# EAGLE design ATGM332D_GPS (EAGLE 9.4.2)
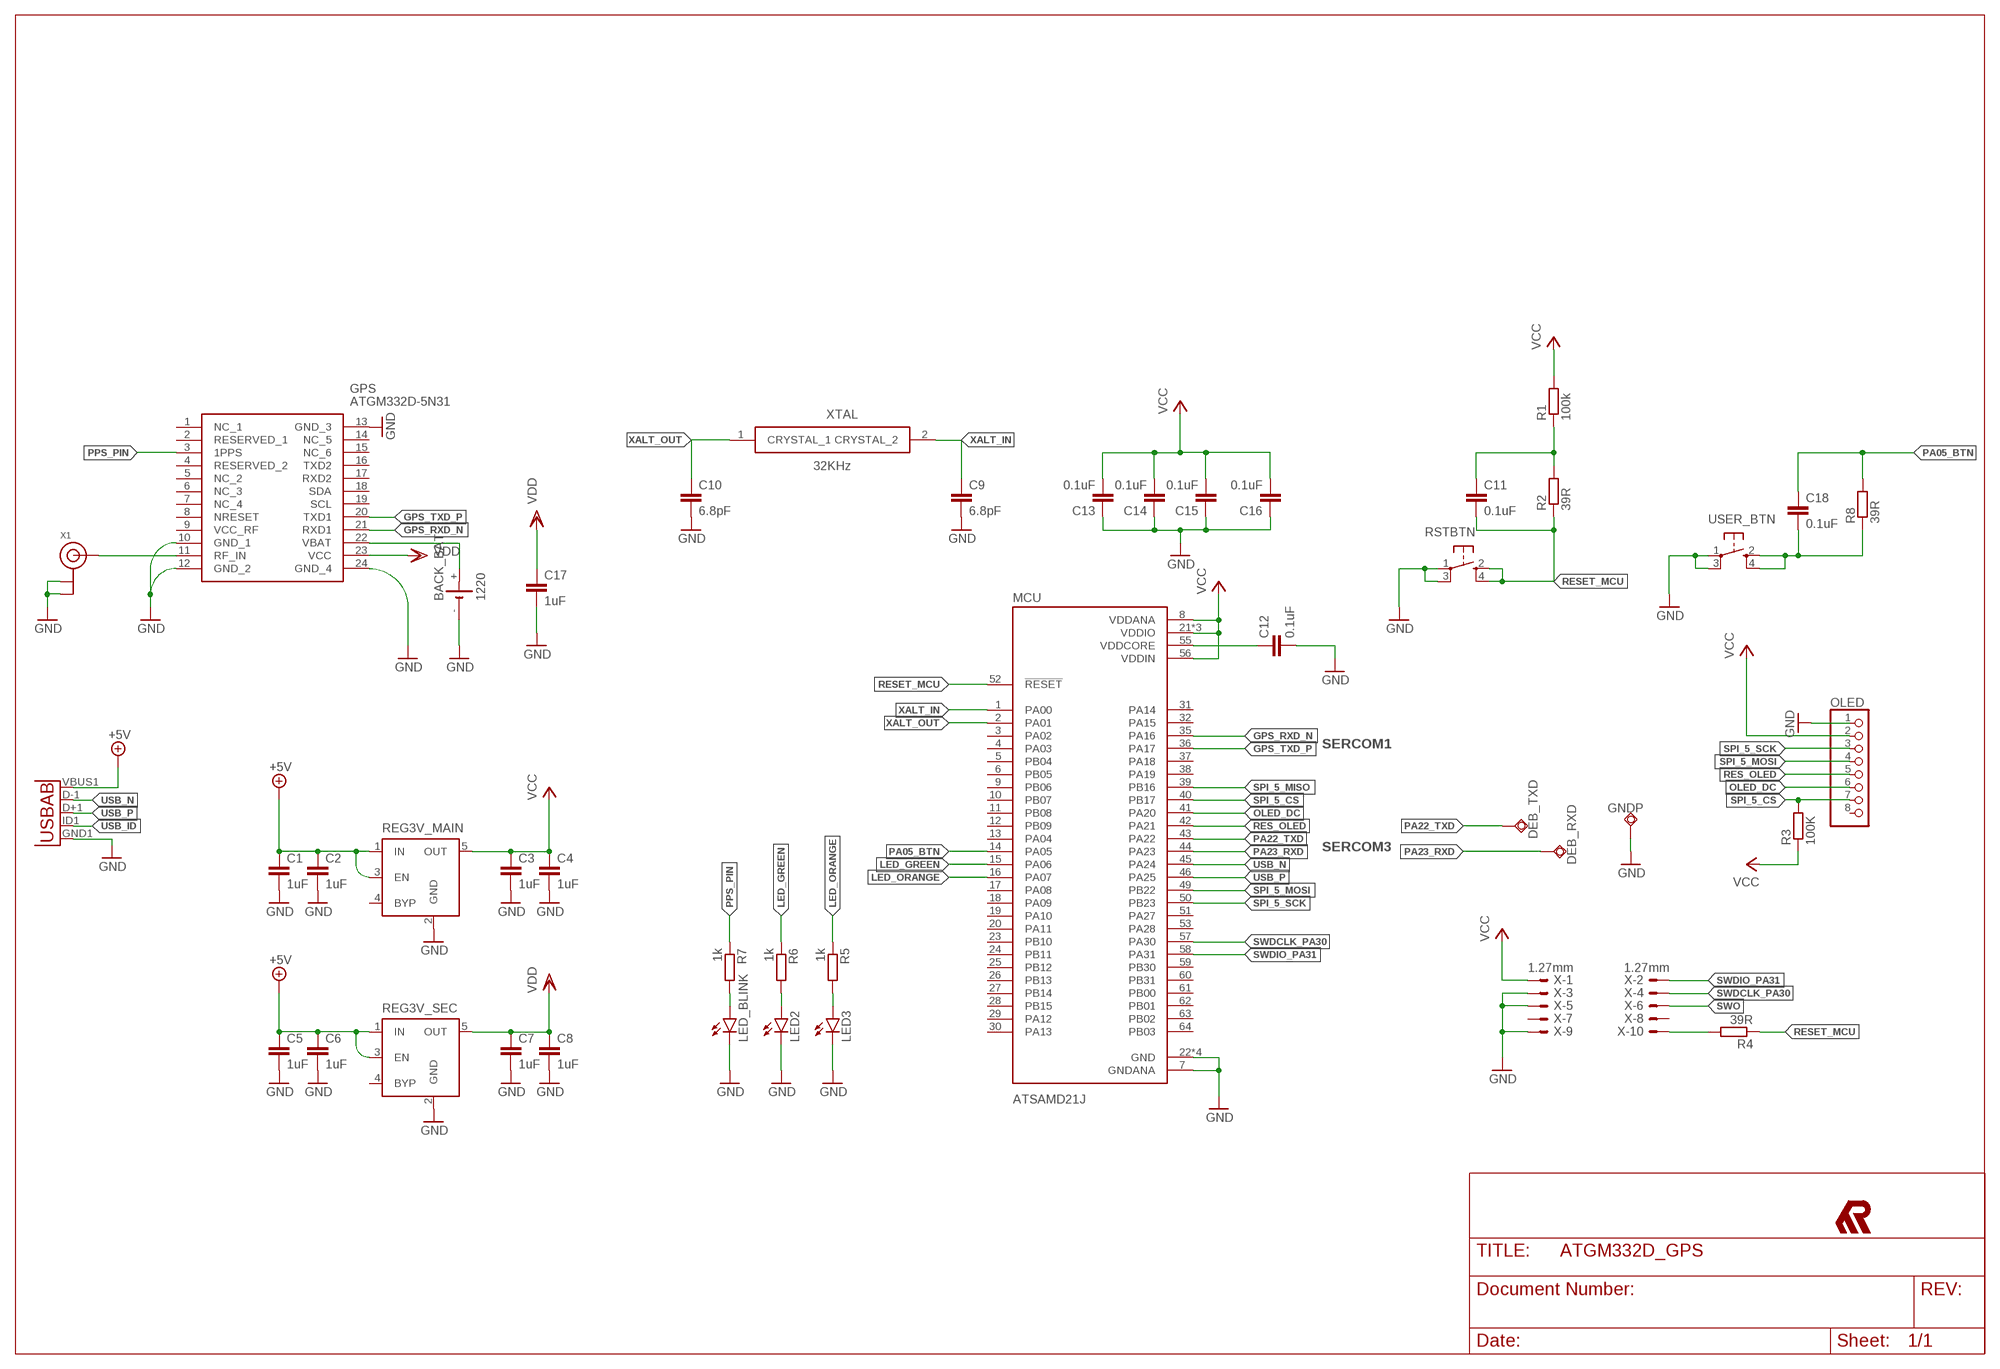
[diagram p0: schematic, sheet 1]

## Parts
BACK_BAT  1220  CH291-1220LF  [CH291-1220LF]
C1  1uF  C-EUC0805  [C0805]
C2  1uF  C-EUC0805  [C0805]
C3  1uF  C-EUC0805  [C0805]
C4  1uF  C-EUC0805  [C0805]
C5  1uF  C-EUC0805  [C0805]
C6  1uF  C-EUC0805  [C0805]
C7  1uF  C-EUC0805  [C0805]
C8  1uF  C-EUC0805  [C0805]
C9  6.8pF  C-EUC0603  [C0603]
C10  6.8pF  C-EUC0603  [C0603]
C11  0.1uF  C-EUC0603  [C0603]
C12  0.1uF  C-EUC0603  [C0603]
C13  0.1uF  C-EUC0603  [C0603]
C14  0.1uF  C-EUC0603  [C0603]
C15  0.1uF  C-EUC0603  [C0603]
C16  0.1uF  C-EUC0603  [C0603]
C17  1uF  C-EUC0805  [C0805]
C18  0.1uF  C-EUC0603  [C0603]
DEB_RXD  TPSQTP18R  [TP18R]
DEB_TXD  TPSQTP18R  [TP18R]
GNDP  TPSQTP18R  [TP18R]
GPS  ATGM332D-5N31  [ATGM332D5N31]
LED2  LEDCHIP-LED0603  [CHIP-LED0603]
LED3  LEDCHIP-LED0603  [CHIP-LED0603]
LED_BLINK  LEDCHIP-LED0603  [CHIP-LED0603]
MCU  ATSAMD21J  ATSAMD21J18A-AU  [QFP80P1600X1600X120-64N]
OLED  PINHD-1X8  [1X08]
R1  100k  R-EU_R0603  [R0603]
R2  39R  R-EU_R0603  [R0603]
R3  100K  R-EU_R0603  [R0603]
R4  39R  R-EU_R0603  [R0603]
R5  1k  R-EU_R0603  [R0603]
R6  1k  R-EU_R0603  [R0603]
R7  1k  R-EU_R0603  [R0603]
R8  39R  R-EU_R0603  [R0603]
REG3V_MAIN  MIC5219XX  [SOT23-5]
REG3V_SEC  MIC5219XX  [SOT23-5]
RSTBTN  SPST_TACT-KMR2  [KMR2]
U$2  MR_SMALL_SIZE12  [MR_SMALL_12MM]
USB  MICRO_USB_B  [USB-MICRO-SMD]
USER_BTN  SPST_TACT-KMR2  [KMR2]
X  1.27mm  1365-10  [1365-10]
X1  ANTENNA_U.FL  [U.FL]
XTAL  32KHz  SMD-3215_2P32.768KHZ12.5PF10PP  [SMD3215_2P32768KHZ125PF10PPM]

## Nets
+5V: C1.1 C2.1 C5.1 C6.1 REG3V_MAIN.1(IN) REG3V_MAIN.3(EN) REG3V_SEC.1(IN) REG3V_SEC.3(EN) USB.VBUS1(VBUS)
GND: BACK_BAT.- C1.2 C2.2 C3.2 C4.2 C5.2 C6.2 C7.2 C8.2 C9.2 C10.2 C12.2 C13.1 C14.1 C15.1 C16.1 C17.2 GNDP.TP GPS.10(GND_1) GPS.12(GND_2) GPS.13(GND_3) GPS.24(GND_4) LED2.C LED3.C LED_BLINK.C MCU.7(GNDANA) MCU.22(GND) MCU.33(GND) MCU.47(GND) MCU.54(GND) OLED.1 REG3V_MAIN.2(GND) REG3V_SEC.2(GND) RSTBTN.1(P) RSTBTN.3(P1) USB.GND1(GND) USER_BTN.1(P) USER_BTN.3(P1) X1.1(GND) X1.2(GND) X.3 X.5 X.9
GPS_RXD_N: GPS.21(RXD1) MCU.35(PA16)
GPS_TXD_P: GPS.20(TXD1) MCU.36(PA17)
LED_GREEN: MCU.15(PA06) R6.1
LED_ORANGE: MCU.16(PA07) R5.1
N$1: R4.2 X.10
N$2: LED_BLINK.A R7.2
N$3: LED2.A R6.2
N$4: LED3.A R5.2
N$5: C18.2 R8.1 USER_BTN.2(S) USER_BTN.4(S1)
N$8: BACK_BAT.+ GPS.22(VBAT)
N$9: GPS.11(RF_IN) X1.3(SIGNAL)
N$10: C11.1 R1.1 R2.2
OLED_DC: MCU.41(PA20) OLED.6
PA05_BTN: C18.1 MCU.14(PA05) R8.2
PA22_TXD: DEB_TXD.TP MCU.43(PA22)
PA23_RXD: DEB_RXD.TP MCU.44(PA23)
PPS_PIN: GPS.3(1PPS) R7.1
RES_OLED: MCU.42(PA21) OLED.5
RESET_MCU: C11.2 MCU.52(!RESET) R2.1 R4.1 RSTBTN.2(S) RSTBTN.4(S1)
SPI_5_CS: MCU.40(PB17) OLED.7 R3.2
SPI_5_MISO: MCU.39(PB16)
SPI_5_MOSI: MCU.49(PB22) OLED.4
SPI_5_SCK: MCU.50(PB23) OLED.3
SWDCLK_PA30: MCU.57(PA30) X.4
SWDIO_PA31: MCU.58(PA31) X.2
SWO: X.6
USB_ID: USB.ID1(USBID)
USB_N: MCU.45(PA24) USB.D-1(D-)
USB_P: MCU.46(PA25) USB.D+1(D+)
VCC: C3.1 C4.1 C13.2 C14.2 C15.2 C16.2 MCU.8(VDDANA) MCU.21(VDDIO) MCU.34(VDDIO) MCU.48(VDDIO) MCU.56(VDDIN) OLED.2 R1.2 R3.1 REG3V_MAIN.5(OUT) X.1
VCORE: C12.1 MCU.55(VDDCORE)
VDD: C7.1 C8.1 C17.1 GPS.23(VCC) REG3V_SEC.5(OUT)
XALT_IN: C9.1 MCU.1(PA00) XTAL.2(CRYSTAL_2)
XALT_OUT: C10.1 MCU.2(PA01) XTAL.1(CRYSTAL_1)
Unconnected: GPS.1(NC_1) GPS.2(RESERVED_1) GPS.4(RESERVED_2) GPS.5(NC_2) GPS.6(NC_3) GPS.7(NC_4) GPS.8(NRESET) GPS.9(VCC_RF) GPS.14(NC_5) GPS.15(NC_6) GPS.16(TXD2) GPS.17(RXD2) GPS.18(SDA) GPS.19(SCL) MCU.3(PA02) MCU.4(PA03) MCU.5(PB04) MCU.6(PB05) MCU.9(PB06) MCU.10(PB07) MCU.11(PB08) MCU.12(PB09) MCU.13(PA04) MCU.17(PA08) MCU.18(PA09) MCU.19(PA10) MCU.20(PA11) MCU.23(PB10) MCU.24(PB11) MCU.25(PB12) MCU.26(PB13) MCU.27(PB14) MCU.28(PB15) MCU.29(PA12) MCU.30(PA13) MCU.31(PA14) MCU.32(PA15) MCU.37(PA18) MCU.38(PA19) MCU.51(PA27) MCU.53(PA28) MCU.59(PB30) MCU.60(PB31) MCU.61(PB00) MCU.62(PB01) MCU.63(PB02) MCU.64(PB03) OLED.8 REG3V_MAIN.4(BYP) REG3V_SEC.4(BYP) X.7 X.8

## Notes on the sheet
- SERCOM1
- SERCOM3

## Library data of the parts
BACK_BAT = battery:CH291-1220LF: Battery Holder, SMT, 12mm
C1-C18 = rcl:C-EU: CAPACITOR, European symbol; SPICEPREFIX: C
DEB_RXD DEB_TXD GNDP = testpad:TPSQ: Test pad
GPS = ATGM332D-5N31:ATGM332D-5N31: Communication Modules/GNSS Modules 12.2x16x2.4mm Source: Datasheet; DESCRIPTION: Communication Modules/GNSS Modules 12.2x16x2.4mm; HEIGHT: 2.6mm; MANUFACTURER_NAME: ZHONGKEWEI; MANUFACTURER_PART_NUMBER: ATGM332D-5N31
LED2 LED3 LED_BLINK = led:LED: LED
MCU = ATSAMD21J18A-AU:ATSAMD21J18A-AU: 256kB Flash, 32kB SRAM, SERCOM, USB - 64TQFP IND TEMP, GREEN, 1.6-3.6V, 48MHz/ TQFP (A); DESCRIPTION: SAMD21J Series 256 kB Flash 32 kB RAM 48 MHz 32-Bit Microcontroller - TQFP-64; DIGI-KEY_PART_NUMBER: ATSAMD21J18A-AU-ND; DIGI-KEY_PURCHASE_URL: https://www.digikey.com/product-detail/en/microchip-technology/ATSAMD21J18A-AU/ATSAMD21J18A-AU-ND/4935901?utm_source=snapeda&utm_medium=aggregator&utm_campaign=symbol; MF: Microchip; MP: ATSAMD21J18A-AU; PACKAGE: TQFP-64 Microchip
OLED = pinhead:PINHD-1X8: PIN HEADER
R1-R8 = rcl:R-EU_: RESISTOR, European symbol; SPICEPREFIX: R
REG3V_MAIN REG3V_SEC = v-reg-micrel:MIC5219XX: VOLTAGE REGULATOR; OC_FARNELL: unknown; OC_NEWARK: unknown
RSTBTN USER_BTN = adafruit:SPST_TACT: SMT 6mm switch, EVQQ2 series http://www.ladyada.net/library/eagle
U$2 = Rawashdeh_Eagle_Logo:MR_SMALL_SIZE: MR Mohannad Rawashdeh Logo 7,12 mm
USB = Rawashdeh_Eagle_Connector:MICRO_USB_B: USB - micro B USB 2.0 Receptacle Connector 5 Position Surface Mount, Right Angle; Through Hole Manf. # 10118194-0001LF
X = con-leotronics:1365-10: DUAL ROW STRAIGHT HEADER 1364 SERIES. 1.27mm x 1.27mm. Without Fixing Post. SMT Source: http://www.leotronics.co.uk/Conexcon/Data%20Sheets/sec.%20A/1364ing.pdf; OC_FARNELL: unknown; OC_NEWARK: unknown
X1 = adafruit:ANTENNA_U.FL: U.FL Antenna Connector
XTAL = SMD-3215_2P32.768KHZ12.5PF10PP:SMD-3215_2P32.768KHZ12.5PF10PP: SMD Crystal Resonators 32.768KHz +/-10ppm SMD-3215_2P RoHS; DESCRIPTION: SMD Crystal Resonators 32.768KHz +/-10ppm SMD-3215_2P RoHS; HEIGHT: 0.8mm; LCSC_PART_NUMBER: C164062; LCSC_PRICE-STOCK: https://lcsc.com/product-detail/SMD-Crystal-Resonators_Zhejiang-Abel-Elec-SMD-3215-2P32-768KHZ12-5PF10PPM_C164062.html; MANUFACTURER_NAME: Zhejiang Abel Elec; MANUFACTURER_PART_NUMBER: SMD-3215_2P32.768KHZ12.5PF10PPM

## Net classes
1 VCC: width 0.203 mm, clearance 0.152 mm
2 VDD: width 0.203 mm, clearance 0.152 mm

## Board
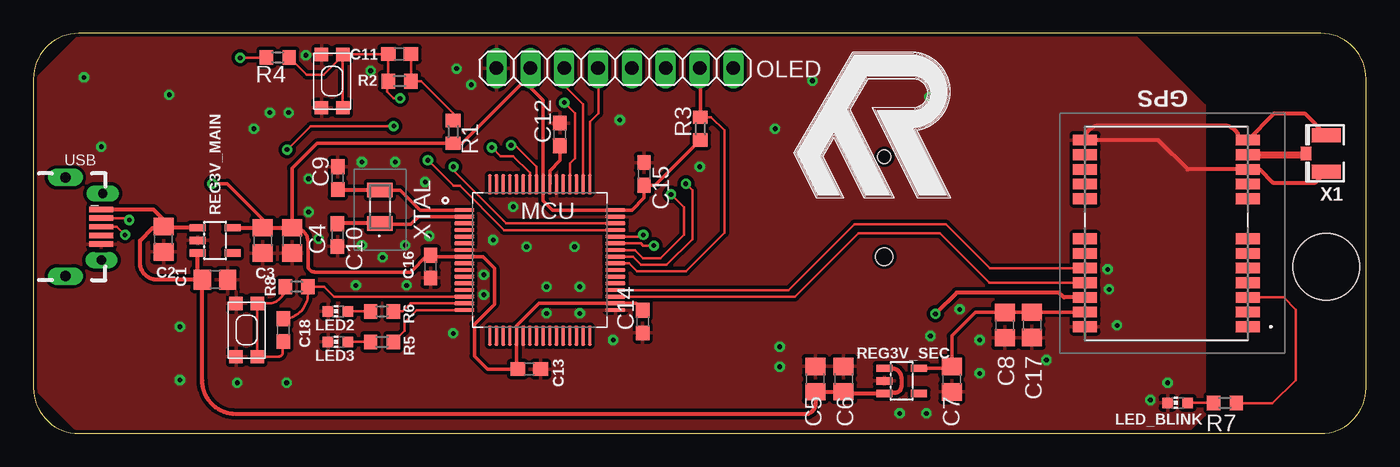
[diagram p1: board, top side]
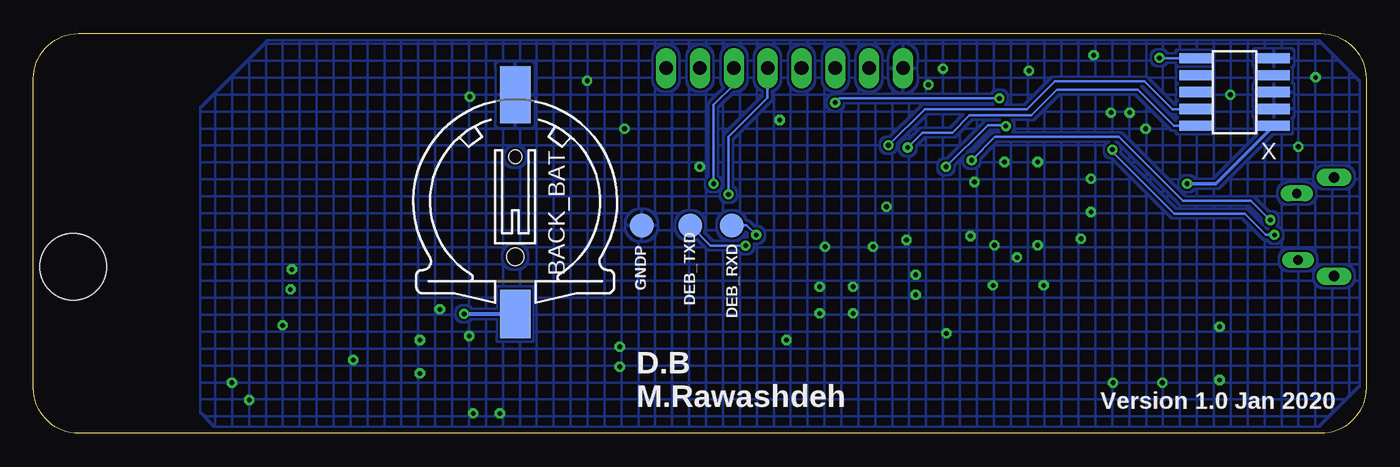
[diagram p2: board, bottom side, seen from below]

Size 100 x 30 mm. Coordinates in mm from the lower left corner, seen from the top.
Outline: 0,26.59 0,3.41 arc90 3.41,0 96.59,0 arc90 100,3.41 100,26.59 arc90 96.59,30 3.41,30 arc90 0,26.59
Copper layers (1*16): Top 0.035mm / dielectric 1.5mm / Bottom 0.035mm
Design rules "default *": minimum track width 6mil, minimum drill 0.35mm, track to track 6mil, track to pad 6mil, pad to pad 6mil, via to via 6mil, smd to smd 6mil, copper to edge 8mil, drill to drill 6mil, minimum pad ring 10mil, minimum via ring 8mil, stop-mask expansion 4mil, vias tented up to drill 0mil, thermal gap 10mil
Holes 5 mm at 97,12.5

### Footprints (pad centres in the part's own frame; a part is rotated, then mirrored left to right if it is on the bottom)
CH291-1220LF = smd 2.3 x 3.66: + 0,-2.296 | smd 2.3 x 4.3: - 0,14.146 | hole 1.3: 0,2 | hole 1: 0,9.5
C0805 = smd 1.3 x 1.5: 1 -0.95,0; 2 0.95,0
C0603 = smd 1.1 x 1: 1 -0.85,0; 2 0.85,0
TP18R = smd 1.8 x 1.8: TP 0,0
ATGM332D5N31 = smd 1.8 x 0.8: 1 6.1,-7; 2 6.1,-5.9; 3 6.1,-4.8; 4 6.1,-3.7; 5 6.1,-2.6; 6 6.1,-1.5; 7 6.1,-0.4; 8 6.1,2.6; 9 6.1,3.7; 10 6.1,4.8; 11 6.1,5.9; 12 6.1,7; 13 -6.1,7; 14 -6.1,5.9; 15 -6.1,4.8; 16 -6.1,3.7; 17 -6.1,2.6; 18 -6.1,-0.4; 19 -6.1,-1.5; 20 -6.1,-2.6; 21 -6.1,-3.7; 22 -6.1,-4.8; 23 -6.1,-5.9; 24 -6.1,-7
CHIP-LED0603 = smd 0.8 x 0.8: A 0,-0.75; C 0,0.75
QFP80P1600X1600X120-64N = smd 1.49 x 0.28: 1 -5.67,3.75; 2 -5.67,3.25; 3 -5.67,2.75; 4 -5.67,2.25; 5 -5.67,1.75; 6 -5.67,1.25; 7 -5.67,0.75; 8 -5.67,0.25; 9 -5.67,-0.25; 10 -5.67,-0.75; 11 -5.67,-1.25; 12 -5.67,-1.75; 13 -5.67,-2.25; 14 -5.67,-2.75; 15 -5.67,-3.25; 16 -5.67,-3.75; 33 5.67,-3.75; 34 5.67,-3.25; 35 5.67,-2.75; 36 5.67,-2.25; 37 5.67,-1.75; 38 5.67,-1.25; 39 5.67,-0.75; 40 5.67,-0.25; 41 5.67,0.25; 42 5.67,0.75; 43 5.67,1.25; 44 5.67,1.75; 45 5.67,2.25; 46 5.67,2.75; 47 5.67,3.25; 48 5.67,3.75 | smd 0.28 x 1.49: 17 -3.75,-5.67; 18 -3.25,-5.67; 19 -2.75,-5.67; 20 -2.25,-5.67; 21 -1.75,-5.67; 22 -1.25,-5.67; 23 -0.75,-5.67; 24 -0.25,-5.67; 25 0.25,-5.67; 26 0.75,-5.67; 27 1.25,-5.67; 28 1.75,-5.67; 29 2.25,-5.67; 30 2.75,-5.67; 31 3.25,-5.67; 32 3.75,-5.67; 49 3.75,5.67; 50 3.25,5.67; 51 2.75,5.67; 52 2.25,5.67; 53 1.75,5.67; 54 1.25,5.67; 55 0.75,5.67; 56 0.25,5.67; 57 -0.25,5.67; 58 -0.75,5.67; 59 -1.25,5.67; 60 -1.75,5.67; 61 -2.25,5.67; 62 -2.75,5.67; 63 -3.25,5.67; 64 -3.75,5.67
1X08 = drill 1.016 long: 1 -8.89,0; 2 -6.35,0; 3 -3.81,0; 4 -1.27,0; 5 1.27,0; 6 3.81,0; 7 6.35,0; 8 8.89,0
R0603 = smd 1 x 1.1: 1 -0.85,0; 2 0.85,0
SOT23-5 = smd 0.55 x 1.2: 1 -0.95,-1.3; 2 0,-1.3; 3 0.95,-1.3; 4 0.95,1.3; 5 -0.95,1.3
KMR2 = smd 1 x 1: 1 2,0.8; 2 2,-0.8; 3 -2,0.8; 4 -2,-0.8
USB-MICRO-SMD = smd 1.8 x 0.4: D+1 2.7,0; D-1 2.7,0.65; GND1 2.7,-1.3; ID1 2.7,-0.65; VBUS1 2.7,1.3 | drill 0.7 pad 0.813 long: H1 2.7,-2.5; H2 2.8,2.5 | drill 0.8 pad 1.016 long: H3 0,-3.7; H4 0,3.7
1365-10 = smd 0.76 x 2.4: 1 -2.54,-2.95; 2 -2.54,2.95; 3 -1.27,-2.95; 4 -1.27,2.95; 5 0,-2.95; 6 0,2.95; 7 1.27,-2.95; 8 1.27,2.95; 9 2.54,-2.95; 10 2.54,2.95
U.FL = smd 2.2 x 1.05: 1 0,1.375; 2 0,-1.375 | smd 0.8 x 1: 3 1.525,0
SMD3215_2P32768KHZ125PF10PPM = smd 1.1 x 1.9: 1 -1.25,0; 2 1.25,0

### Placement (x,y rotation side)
BACK_BAT  63.85,11.25 0 bottom
C1  13.63,11.53 0 top
C2  9.77,14.56 270 top
C3  17.21,14.47 270 top
C4  19.4,14.47 270 top
C5  58.67,4.07 90 top
C6  60.79,4.07 90 top
C7  68.91,4.05 270 top
C8  72.88,8.12 270 top
C9  22.84,19.14 90 top
C10  22.82,14.87 270 top
C11  27.48,28.44 180 top
C12  39.5,22.42 90 top
C13  37.2,4.82 180 top
C14  45.72,8.38 90 top
C15  45.82,19.45 270 top
C16  29.81,12.51 90 top
C17  74.93,8.13 270 top
C18  18.75,7.75 270 top
DEB_RXD  47.59,15.6 0 bottom
DEB_TXD  50.71,15.6 0 bottom
GNDP  54.36,15.6 0 bottom
GPS  85,15 0 top
LED2  22.86,9.14 90 top
LED3  22.86,6.86 90 top
LED_BLINK  85.85,2.29 90 top
MCU  38,13 0 top
OLED  43.64,27.38 0 top
R1  31.5,22.61 270 top
R2  27.48,26.41 0 top
R3  50.04,22.86 90 top
R4  18.35,28.19 180 top
R5  26.16,6.86 180 top
R6  26.16,9.14 180 top
R7  89.41,2.29 180 top
R8  19.75,11 0 top
REG3V_MAIN  13.64,14.46 270 top
REG3V_SEC  65.15,3.93 270 top
RSTBTN  22.42,26.42 90 top
U$2  64.05,21 0 top
USB  2.41,15.5 0 top
USER_BTN  16,7.75 90 top
X  9.88,25.6 90 bottom
X1  97,21 180 top
XTAL  26,17 90 top

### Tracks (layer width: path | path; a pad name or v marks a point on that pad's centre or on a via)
+5V
  Top 0.305: REG3V_MAIN.1 9.86,15.41 | 9.86,15.41 C2.1 9.77,16.03 9,16.8 USB.VBUS1 | C1.1 arc-90 12.34,11.86 REG3V_MAIN.3 | C1.1 arc-90 C1.1 12.67,3.98 arc90 15.21,1.44 57.92,1.44 arc90 58.67,2.19 C5.1 C6.1 60.94,2.98 REG3V_SEC.3 arc-90 63.91,3.04 64.64,3.04 arc90 65.12,3.52 65.12,4.16 arc90 64.4,4.88 REG3V_SEC.1 | C1.1 9.27,11.53 arc-90 8,12.8 8,14.45 8.96,15.41 9.86,15.41
GND  (via drill 0.35)
  Top 0.305: X1.2 95.38,24 93.1,24 GPS.12 arc-90 91,21.9 90.5,21.9 arc90 89.3,23.1 80,23.1 arc90 GPS.13 84.4,22 86.6,19.8 GPS.10 92,19.8 93,18.8 96.17,18.8 X1.1
  other vias: 40.6,14 37,14 34.5,14.5 36,17 44,23.5 50,20 41,11 38.5,11 41,9 38.5,9 43.5,7 31.5,7.5 33.8,10.4 33.8,11.9 5.1,21.5 10.2,25.4 3.8,26.7 15.3,3.8 19,3.8 11,8 11,4 56,6.5 56,5 65,1.5 67,1.5 71,4.5 76,5.5 71,7 69.5,9.3 67.3,7.3 80.6,12.3 80.7,10.8 81.3,8.1 83.8,2.5 85.1,3.8 29.7,14.8 28,11.1 24.2,11.1 26.2,13.2 24.65,14.1 27.9,14.1 24.65,20.35 27.15,20.35 29.4,18.85 20.65,19.1 20.65,16.6 21.4,14.6 25.3,27.2 20.45,28.35 19.15,24.05 16.55,22.85 17.75,24.05 31.75,27.35 32.85,26.15 58.45,26.45 55.65,22.85 67.25,25.25
  pour Bottom (hatched): 3.5,29.5 82.5,29.5 87.5,24.5 87.5,1.5 86.5,0.5 3.5,0.5 0.5,3.5 0.5,26.5
  pour Top (isolate 0.254): 3.45,29.85 82.65,29.85 87.9,24.6 87.9,1.35 86.7,0.15 3.3,0.15 0.15,3.3 0.15,26.55 0.3,26.7
GPS_RXD_N
  Top 0.203: MCU.35 57.13,10.25 61.9,15.02 68.02,15.02 71.74,11.3 GPS.21
GPS_TXD_P
  Top 0.203: GPS.20 71.76,12.4 68.48,15.68 61.6,15.68 56.67,10.75 MCU.36
LED_GREEN
  Top 0.203: MCU.15 28.31,9.75 27.7,9.14 R6.1
LED_ORANGE
  Top 0.203: MCU.16 28.77,9.25 27.84,8.32 27.84,7.68 R5.1
N$1  (via drill 0.35)
  Top 0.203: v15.52,28.16 17.46,28.16 R4.2
  Bottom 0.203: X.10 15.5,28.14 v15.52,28.16
N$2
  Top 0.203: LED_BLINK.A R7.2
N$3
  Top 0.203: R6.2 LED2.A
N$4
  Top 0.203: R5.2 LED3.A
N$5
  Top 0.203: USER_BTN.4 16.9,5.75 | 16.9,5.75 18.39,5.75 arc90 18.72,6.08 18.72,6.87 arc-90 C18.2 | R8.1 arc-90 17.65,9.75 USER_BTN.2 16.8,5.85 16.9,5.75
N$8  (via drill 0.35)
  Top 0.305: GPS.22 77.32,10.2 76.96,10.56 69.28,10.56 v67.68,8.96
  Bottom 0.305: v67.68,8.96 BACK_BAT.+
N$9
  Top 0.508: GPS.11 95.38,20.9 X1.3
N$10
  Top 0.203: C11.1 R2.2 29.11,26.41 31.5,24.02 R1.1
OLED_DC  (via drill 0.35)
  Top 0.203: MCU.41 44.99,13.25 45.6,12.64 47.52,12.64 49.44,14.56 49.44,18.24 v48.96,18.72
  Bottom 0.203: v48.96,18.72 48.96,24.64 47.45,26.15 OLED.6
PA05_BTN
  Top 0.203: MCU.14 22.55,10.25 21.8,11 R8.2 20.6,10.45 arc-90 C18.1
PA22_TXD  (via drill 0.35)
  Top 0.203: MCU.43 45.5,14.25 45.59,14.25 45.76,14.08 v46.56,14.08
  Bottom 0.203: v46.56,14.08 49.19,14.08 DEB_TXD.TP
PA23_RXD  (via drill 0.35)
  Top 0.203: MCU.44 45.63,14.75 v45.76,14.88
  Bottom 0.203: v45.76,14.88 46.48,15.6 DEB_RXD.TP
PPS_PIN
  Top 0.203: GPS.3 93.8,10.2 94.72,9.28 94.72,4 92.96,2.24 90.3,2.24 R7.1
RES_OLED  (via drill 0.35)
  Top 0.203: MCU.42 45.13,13.75 45.76,13.12 47.04,13.12 48.8,14.88 48.8,16.96 v47.84,17.92
  Bottom 0.203: v47.84,17.92 47.84,22.24 44.91,25.17 OLED.5
RESET_MCU  (via drill 0.35)
  Top 0.203: 23.22,28.32 RSTBTN.2 26.6,28.42 C11.2 R2.1 26.56,26.34 26.56,25.6 27.04,25.12 v27.52,25.12 | 23.22,28.32 RSTBTN.4 | R4.1 20.51,26.88 21.78,26.88 23.22,28.32 | MCU.52 40.25,20.25 40.64,20.64 40.64,24 v39.84,24.8
  Bottom 0.203: v39.84,24.8 39.52,25.12 v27.52,25.12
SPI_5_CS
  Top 0.203: R3.2 50.85,23.71 51.84,22.72 51.84,15.04 48.96,12.16 45.28,12.16 44.69,12.75 MCU.40
  Top 0.254: R3.2 50.04,27.33 OLED.7
SPI_5_MOSI
  Top 0.203: MCU.49 41.75,23.35 42.4,24 42.4,27.35 OLED.4
SPI_5_SCK
  Top 0.203: MCU.50 41.25,24.67 39.83,26.09 OLED.3
SWDCLK_PA30  (via drill 0.35)
  Top 0.203: v35.84,21.6 36.16,21.6 37.75,20.01 MCU.57
  Bottom 0.203: v35.84,21.6 33.12,24.32 25.44,24.32 23.36,26.4 16.64,26.4 14.56,24.32 12.84,24.32 X.4
SWDIO_PA31  (via drill 0.35)
  Top 0.203: MCU.58 37.25,19.55 36,20.8 35.04,20.8 v34.4,21.44
  Bottom 0.203: X.2 14.42,23.06 17.12,25.76 23.2,25.76 25.12,23.84 29.76,23.84 31.04,22.56 33.28,22.56 v34.4,21.44
USB_N  (via drill 0.35)
  Top 0.203: USB.D-1 7.05,16.15 v7.2,16 | MCU.45 35.31,15.25 32,18.56 31.52,18.56 v29.6,20.48
  Bottom 0.203: v7.2,16 8.64,17.44 13.76,17.44 18.56,22.24 27.84,22.24 v29.6,20.48
USB_P  (via drill 0.35)
  Top 0.203: USB.D+1 6.26,15.5 v6.88,14.88 | MCU.46 35.45,15.75 31.52,19.68 v31.52,20 | v19.04,21.28 20.8,23.04 v27.04,23.04
  Bottom 0.203: v6.88,14.88 7.52,14.88 9.12,16.48 14.4,16.48 19.04,21.12 v19.04,21.28 | v31.52,20 28.4,23.12 27.12,23.12 v27.04,23.04
VCC  (via drill 0.35)
  Top 0.254: C14.2 45.2,9.75 MCU.34 37.93,9.75 36.25,8.07 MCU.21 36.25,4.92 C13.2 34.08,4.82 33.1,5.8 33.1,8.2 34.6,9.7 34.6,12.4 33.75,13.25 MCU.8 29.92,13.25 C16.2 29.56,13.36 28.3,12.1 21.1,12.1 arc-90 20.6,12.6 20.6,14.4 arc90 19.58,15.42 C4.1 19.4,19.88 21.28,21.76 R1.2 32.16,21.76 37.29,26.88 | R3.1 46.63,18.6 C15.2 45.82,17.66 44.91,16.75 MCU.48 38.95,16.75 38.25,17.45 MCU.56 38.25,24.97 37.29,25.93 37.29,26.88 | 37.29,26.88 OLED.2 | v13.44,18.72 14.56,18.72 17.21,16.07 C3.1
  Top 0.305: REG3V_MAIN.5 C3.1 arc90 C3.1 C4.1
  Bottom 0.254: X.1 11.27,18.72 v13.44,18.72
VCORE
  Top 0.254: MCU.55 38.75,19.71 39.52,20.48 39.52,21.55 C12.1
VDD
  Top 0.254: GPS.23 74.95,9.1 C17.1 C8.1 70.67,9.07 68.91,7.31 C7.1 68.78,4.88 REG3V_SEC.5
XALT_IN
  Top 0.254: MCU.1 29.01,16.75 27.51,18.25 XTAL.2
  Top 0.305: XTAL.2 22.88,18.25 C9.1
XALT_OUT
  Top 0.254: MCU.2 28.89,16.25 28.32,15.68 26.07,15.68 XTAL.1
  Top 0.305: XTAL.1 22.85,15.75 C10.1

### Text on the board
bNames: Version 1.0 Jan 2020 | D.B / M.Rawashdeh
